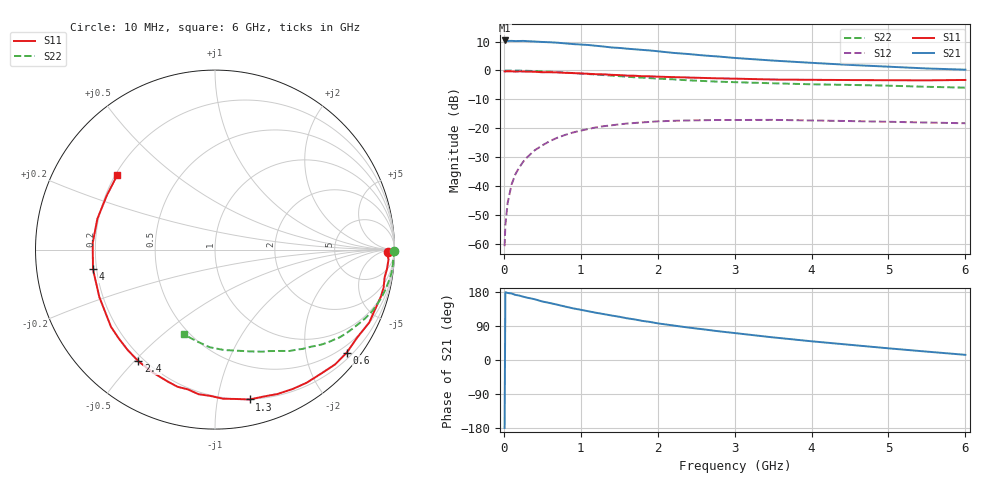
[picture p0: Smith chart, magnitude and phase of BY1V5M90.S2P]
! SIEMENS Small Signal Semiconductors
! BFY420
! Si NPN RF SIEGET Grounded Emitter Transistor in MICRO-X
! VCE = 1.5 V  IC = 0.9 mA
! Common Emitter S-Parameters:  October  1996
# GHz  S  MA  R  50
!  f  S11  S21  S12  S22
! GHz  MAG  ANG  MAG  ANG  MAG  ANG  MAG  ANG
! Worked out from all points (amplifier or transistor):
!   36 points, 10 MHz to 6 GHz, reference 50 ohm
!   highest |S21| = 10.4 dB at 10 MHz (marker M1)
!   |S21| within 3 dB of that: start of sweep to 1.672 GHz
!   unconditionally stable (mu >= 1): 4.611 GHz to end of sweep
!   at 250 MHz: K = 0.04, MSG = 21.0 dB, |S12| = -31.7 dB
!   at 1.4 GHz: K = 0.21, MSG = 13.5 dB, |S12| = -19.0 dB
!   at 6 GHz: K = 1.33, MAG = 5.8 dB, |S12| = -18.3 dB
!   S11 on the Smith chart (normalised r, x): 10 MHz: 48, -16; 600 MHz: 0.33, -2.87; 1.3 GHz: 0.20, -1.24; 2.4 GHz: 0.18, -0.51; 4 GHz: 0.19, -0.08; 6 GHz: 0.21, +0.33
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0.01  0.9631 -0.7  3.313 -179.3  0.0009 88.9  0.9989 -0.3
0.02  0.9585 -1.5  3.279 178.8  0.0021 101.7  0.9911 -0.7
0.05  0.9685 -3.2  3.244 176.9  0.0051 86.0  0.9975 -1.6
0.1  0.9644 -6.3  3.258 175.5  0.0105 86.8  0.9945 -3.2
0.15  0.9577 -9.4  3.231 171.8  0.0159 83.5  0.9944 -4.9
0.2  0.963 -12.7  3.241 170.1  0.0208 81.9  0.9934 -6.5
0.3  0.9541 -19.0  3.225 164.6  0.031 79.1  0.9859 -9.7
0.4  0.9504 -25.3  3.175 160.4  0.0412 74.8  0.977 -12.9
0.5  0.9315 -31.7  3.118 154.4  0.0503 70.5  0.9652 -16.1
0.6  0.932 -38.0  3.084 150.3  0.0599 66.6  0.9518 -19.1
0.8  0.9094 -49.4  2.946 140.9  0.0766 59.3  0.9189 -24.8
1.1  0.8766 -66.6  2.764 128.6  0.0969 49.1  0.8668 -32.6
1.3  0.8571 -77.0  2.599 121.1  0.1082 43.1  0.8316 -37.1
1.8  0.7936 -100.9  2.272 103.2  0.1259 30.2  0.75 -46.8
2.2  0.7672 -117.2  2.018 91.2  0.1341 21.6  0.7018 -53.6
2.4  0.7541 -124.5  1.927 85.6  0.136 18.3  0.6748 -56.8
2.8  0.7293 -137.6  1.741 75.6  0.1386 12.1  0.6382 -62.4
3.5  0.6966 -157.7  1.484 59.7  0.1391 3.8  0.5991 -71.2
4  0.6886 -170.8  1.356 49.4  0.136 -0.7  0.5759 -77.9
4.5  0.6824 176.9  1.248 40.1  0.1327 -4.4  0.5617 -84.9
5.5  0.674 153.3  1.083 22.1  0.1251 -8.0  0.521 -101.1
6  0.685 142.6  1.032 13.6  0.1216 -8.0  0.5034 -110.4
